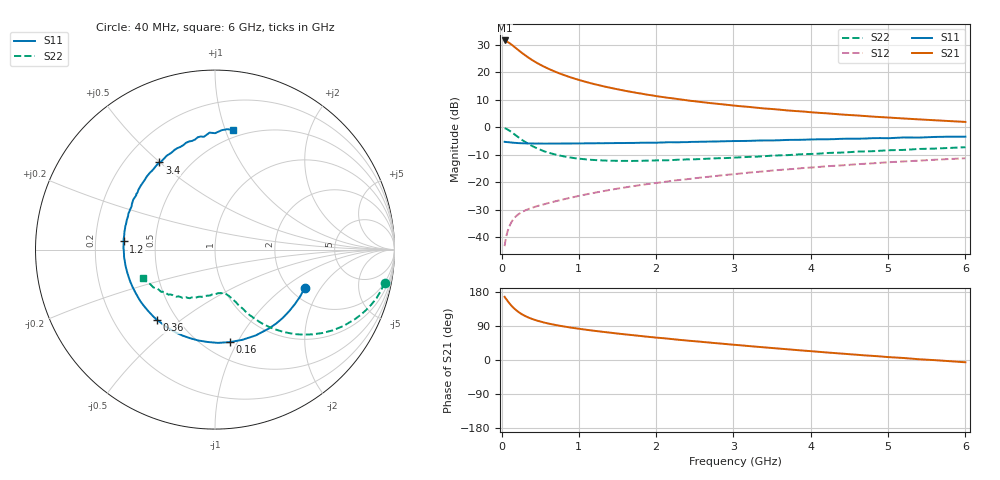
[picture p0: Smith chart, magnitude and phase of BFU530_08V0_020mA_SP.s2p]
! Filename:  P:\Prog\Test\Noise\ATS_data\Testdata_Net\03 Spar\BFU530_APG2013_40_A05_08p0V_020mA_SP_CM01_D.s2p
! Date/Time: Fri 26/Apr/2013 13:03:13
! BFU530_APG2013_40_A05_08p0V_1to25mA_SP_CM01_Bias7_R.s2p
! MDIF S-parameter v. bias file
! BFU530_APG2013_40_A05_08p0V_1to25mA_SP_CM01
! Date/time Wed Apr 24 16:58:28 2013
! VAR V_out= 8.0000
! VAR I_out= 19.9950
! VAR V_in= 0.8172
! VAR I_in= 0.2122
! Device data file deembeded for feedlines and parallel
! Original file: \03 Spar\BFU530_APG2013_40_A05_08p0V_020mA_SP_CM01_R.s2p
! Feed-files: PR047V01_250413_Feed1.s2p, PR047V01_250413_Feed2.s2p
! Parallel-file: PR047V01_250413_Par.s2p
# MHz S MA R 50
!  Freq-MHz  S11-mag  S11-arg  S21-mag  S21-arg  S12-mag  S12-arg  S22-mag  S22-arg
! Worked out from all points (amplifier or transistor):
!   98 points, 40 MHz to 6 GHz, reference 50 ohm
!   highest |S21| = 31.6 dB at 40 MHz (marker M1)
!   |S21| within 3 dB of that: start of sweep to 195.4 MHz
!   unconditionally stable (mu >= 1): 1.361 GHz to 3.557 GHz
!   at 300 MHz: K = 0.46, MSG = 28.3 dB, |S12| = -30.4 dB
!   at 1.6 GHz: K = 1.03, MAG = 16.5 dB, |S12| = -21.9 dB
!   at 6 GHz: K = 0.87, MSG = 6.6 dB, |S12| = -11.3 dB
!   S11 on the Smith chart (normalised r, x): 40 MHz: 2.37, -1.45; 160 MHz: 0.66, -0.93; 360 MHz: 0.39, -0.41; 1.2 GHz: 0.32, +0.04; 3.4 GHz: 0.34, +0.50; 6 GHz: 0.43, +1.06
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40  0.5437 -23.3  38.06 166.8  0.00684 80.6  0.963 -11.1
50  0.5415 -29.1  37.78 163.4  0.008459 78.6  0.9524 -13.9
80  0.5361 -45.2  35.66 155.4  0.01292 72.9  0.9074 -21.7
100  0.5328 -55.2  34.22 150.2  0.01553 69.4  0.8714 -26.4
120  0.5293 -64.6  32.74 145.2  0.01786 66.3  0.8336 -30.6
160  0.5219 -80.9  29.55 136.8  0.02179 61.2  0.7579 -37.8
200  0.5164 -94.4  26.62 129.7  0.02488 57.6  0.6861 -43.7
260  0.5121 -110.7  22.86 121.2  0.02842 54.2  0.5965 -50.2
300  0.5094 -119.2  20.75 116.7  0.03034 52.8  0.5475 -53.6
360  0.5079 -129.7  18.11 111.1  0.03286 51.6  0.4877 -57.5
460  0.5051 -142.6  14.81 104.0  0.03658 51.4  0.4143 -62.0
600  0.5042 -155.5  11.75 96.5  0.04146 52.3  0.3479 -66.0
800  0.5059 -167.9  8.999 88.8  0.04866 54.2  0.2962 -70.2
1050  0.5087 -179.6  6.95 81.0  0.05814 56.1  0.264 -74.4
1200  0.5112 174.9  6.106 77.0  0.06401 56.8  0.2536 -76.9
1600  0.517 162.4  4.608 67.6  0.08028 57.5  0.2442 -83.6
2050  0.527 151.7  3.606 58.2  0.0987 56.8  0.2494 -91.8
3100  0.5623 128.6  2.412 38.6  0.1443 52.4  0.2847 -110.8
3400  0.5757 122.5  2.198 33.3  0.1575 50.4  0.2974 -116.2
4100  0.6031 110.2  1.832 21.7  0.1892 45.5  0.3306 -128.0
5200  0.6524 92.7  1.446 5.3  0.2387 36.5  0.3869 -145.8
6000  0.6742 81.5  1.251 -6.0  0.2727 29.1  0.4333 -158.2
